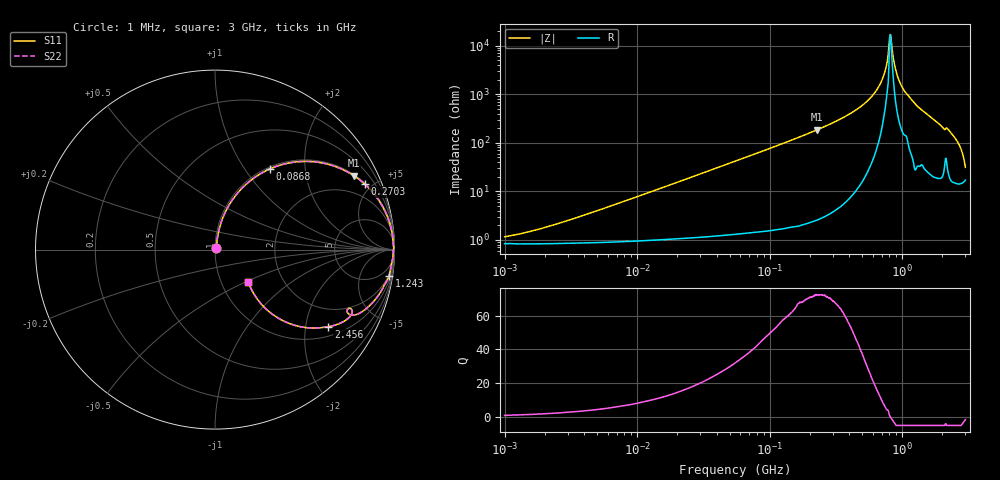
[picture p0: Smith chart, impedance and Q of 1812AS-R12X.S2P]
!s-Parameter Generated by FASTRON Sdn. Bhd.
!FASTRON P/N : 1812AS-R12X
!Keysight Technologies,E4991B,MY54100416,A.01.15
!Date created: Fri Oct 13 14:49:14 2023
!Version  : Rev00 Fri Oct 13 14:49:14 2023
!Data & Calibration Information:
!Freq	S11	S21	S12	S22
!PortZ  Port1:50+j0  Port2:50+j0
!When reading, reference impedance value at option line is always used.
! Remarks : This data is being provided solely for informational purposes.
# Hz S dB R 50
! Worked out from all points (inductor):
!   1601 points, 1 MHz to 3 GHz, reference 50 ohm
!   read as one part in series: L = 124 nH near 3.257 MHz
!   highest Q = 72.3 at 229.1 MHz (marker M1), where L = 129 nH
!   self-resonance near 812.7 MHz
!   S11 on the Smith chart (normalised r, x): 1 MHz: 1.02, +0.02; 86.8 MHz: 1.03, +1.32; 270.3 MHz: 1.06, +4.53; 1.243 GHz: 2, -13; 2.456 GHz: 1.30, -2.68; 3 GHz: 1.34, -0.52
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1000000  -38.81 43.2  -0.07 -0.5  -0.07 -0.5  -38.81 43.2
3804036  -30.26 72.2  -0.08 -1.7  -0.08 -1.7  -30.26 72.2
1.447069e7  -19.22 78.6  -0.14 -6.3  -0.14 -6.3  -19.22 78.6
5.477226e7  -8.42 65.9  -0.79 -22.3  -0.79 -22.3  -8.42 65.9
8.679508e7  -5.27 55.7  -1.66 -33.0  -1.66 -33.0  -5.27 55.7
2.083556e8  -1.39 30.8  -5.83 -58.4  -5.83 -58.4  -1.39 30.8
2.291374e8  -1.15 28.1  -6.54 -61.1  -6.54 -61.1  -1.15 28.1
2.702786e8  -0.82 23.7  -7.92 -65.5  -7.92 -65.5  -0.82 23.7
4.413523e8  -0.24 12.2  -13.51 -76.6  -13.51 -76.6  -0.24 12.2
6.049187e8  -0.09 5.8  -19.89 -81.5  -19.89 -81.5  -0.09 5.8
7.243229e8  -0.05 2.4  -27.67 -80.1  -27.67 -80.1  -0.05 2.4
7.576891e8  -0.05 1.5  -31.43 -76.8  -31.43 -76.8  -0.05 1.5
7.925923e8  -0.03 0.6  -39.47 -67.5  -39.47 -67.5  -0.03 0.6
8.12673e8  -0.05 0.1  -44.67 -10.7  -44.67 -10.7  -0.05 0.1
8.291033e8  -0.05 -0.3  -41.76 41.2  -41.76 41.2  -0.05 -0.3
8.937307e8  -0.06 -1.8  -30.10 76.0  -30.10 76.0  -0.06 -1.8
9.779672e8  -0.09 -3.6  -24.02 79.1  -24.02 79.1  -0.09 -3.6
1.243477e9  -0.16 -8.7  -16.44 78.8  -16.44 78.8  -0.16 -8.7
1.809789e9  -0.74 -19.6  -9.46 66.4  -9.46 66.4  -0.74 -19.6
2.455801e9  -2.34 -34.2  -4.94 49.3  -4.94 49.3  -2.34 -34.2
2.741597e9  -4.68 -44.9  -2.90 35.1  -2.90 35.1  -4.68 -44.9
3e9  -11.71 -44.3  -1.58 12.6  -1.58 12.6  -11.71 -44.3
